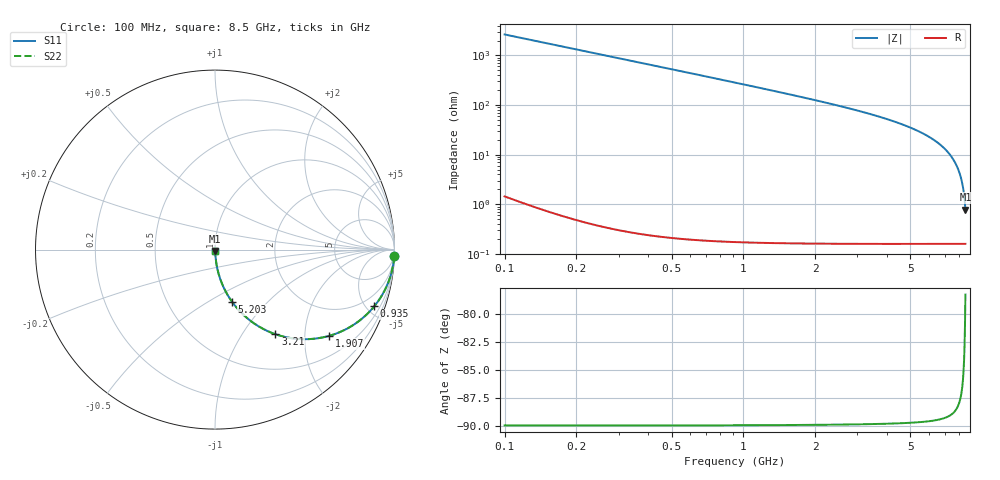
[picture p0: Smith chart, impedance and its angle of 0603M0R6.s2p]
! Created Wed Apr 18 11:57:58 2012
# hz S ma R 50
! 2 Port Network Data from SP1.SP block
! freq  magS11  angS11  magS21  angS21  magS12  angS12  magS22  angS22
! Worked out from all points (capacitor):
!   8401 points, 100 MHz to 8.5 GHz, reference 50 ohm
!   read as one part in series: C = 600 fF near 142 MHz
!   lowest |Z| = 783 mohm at 8.5 GHz (marker M1)
!   S11 on the Smith chart (normalised r, x): 100 MHz: 1, -53; 935 MHz: 1.00, -5.61; 1.907 GHz: 1.00, -2.65; 3.21 GHz: 1.00, -1.42; 5.203 GHz: 1.00, -0.65; 8.5 GHz: 1.00, -0.02
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1e8  0.9993 -2.2  0.03768 87.8  0.03768 87.8  0.9993 -2.2
1.81e8  0.9977 -3.9  0.06811 86.1  0.06811 86.1  0.9977 -3.9
2.33e8  0.9961 -5.0  0.08756 85.0  0.08756 85.0  0.9961 -5.0
3.93e8  0.9891 -8.4  0.1468 81.5  0.1468 81.5  0.9891 -8.4
6.26e8  0.9729 -13.3  0.2308 76.6  0.2308 76.6  0.9729 -13.3
9.35e8  0.9417 -19.6  0.3359 70.3  0.3359 70.3  0.9417 -19.6
1.5e9  0.8635 -30.2  0.5035 59.7  0.5035 59.7  0.8635 -30.2
1.907e9  0.7973 -37.1  0.6027 52.9  0.6027 52.9  0.7973 -37.1
2.9e9  0.6293 -50.9  0.7759 39.0  0.7759 39.0  0.6293 -50.9
3.21e9  0.5792 -54.5  0.8139 35.4  0.8139 35.4  0.5792 -54.5
4.3e9  0.4198 -65.0  0.9062 24.8  0.9062 24.8  0.4198 -65.0
5.203e9  0.3076 -71.8  0.95 17.9  0.95 17.9  0.3076 -71.8
5.7e9  0.2527 -75.0  0.966 14.6  0.966 14.6  0.2527 -75.0
6.479e9  0.1747 -79.4  0.9831 10.1  0.9831 10.1  0.1747 -79.4
7.1e9  0.1185 -82.4  0.9914 6.8  0.9914 6.8  0.1185 -82.4
7.657e9  0.07207 -84.6  0.9958 4.1  0.9958 4.1  0.07207 -84.6
7.875e9  0.05478 -85.2  0.9969 3.1  0.9969 3.1  0.05478 -85.2
8.056e9  0.04078 -85.4  0.9976 2.3  0.9976 2.3  0.04078 -85.4
8.2e9  0.02986 -85.2  0.998 1.7  0.998 1.7  0.02986 -85.2
8.317e9  0.02114 -84.5  0.9982 1.2  0.9982 1.2  0.02114 -84.5
8.401e9  0.01497 -83.0  0.9983 0.9  0.9983 0.9  0.01497 -83.0
8.5e9  0.007815 -77.8  0.9984 0.4  0.9984 0.4  0.007815 -77.8
